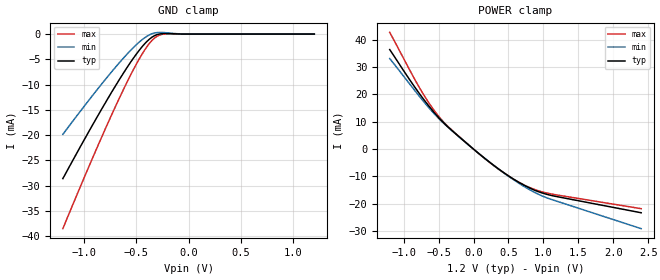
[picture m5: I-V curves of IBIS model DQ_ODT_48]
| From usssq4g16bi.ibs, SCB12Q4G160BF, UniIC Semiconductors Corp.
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|   Model DQ_ODT_48
[Model] DQ_ODT_48
Model_type Input
Polarity   Non-Inverting
Enable   Active-High
Vinl =  8.300E-01
Vinh =  9.700E-01
C_comp   7.893E-13   7.832E-13   8.052E-13
C_comp_power_clamp   2.190E-13   2.022E-13   2.435E-13
C_comp_gnd_clamp   5.703E-13   5.617E-13   5.809E-13
[Model Spec]
Vinh   9.700E-01   9.250E-01   1.015E+00
Vinl   8.300E-01   7.850E-01   8.750E-01
[Temperature Range]   45.000   95.000   -40.000
[Voltage Range]   1.200E+00   1.140E+00   1.260E+00
[C Comp Corner]
C_comp_power_clamp   2.190E-13   2.022E-13   2.435E-13
C_comp_gnd_clamp   5.703E-13   5.809E-13   5.617E-13
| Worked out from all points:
|   GND clamp passes 1 mA (typ) near -0.37 V on its own axis
|   POWER clamp passes 1 mA (typ) near -0.05 V on its own axis
[GND_clamp]
|Voltage   I(typ)   I(min)   I(max)
-1.2V     -28.63mA   -19.87mA   -38.54mA
-875mV    -16.5mA    -11.07mA   -22.57mA
-750mV    -12.06mA   -7.865mA   -16.71mA
-625mV    -7.836mA   -4.834mA   -11.13mA
-525mV    -4.725mA   -2.631mA   -6.977mA
-450mV    -2.664mA   -1.214mA   -4.181mA
-375mV    -1.027mA   -166uA     -1.874mA
-325mV    -315.4uA   217.4uA    -786.6uA
-275mV    28.27uA    334.2uA    -178.9uA
-200mV    103.9uA    241.9uA    49.02uA
-25mV     0A         0A         0A
1.2V      0A         0A         0A
[POWER_clamp]
|Voltage   I(typ)   I(min)   I(max)
-1.2V     36.4mA     33.1mA     42.68mA
-775mV    20.3mA     19.29mA    22.5mA
-625mV    15.29mA    14.69mA    16.38mA
-500mV    11.54mA    11.24mA    12.04mA
-375mV    8.324mA    8.207mA    8.507mA
-125mV    2.721mA    2.687mA    2.776mA
150mV     -3.161mA   -3.14mA    -3.216mA
400mV     -8.009mA   -8.069mA   -8.075mA
575mV     -11mA      -11.23mA   -11mA
725mV     -13.22mA   -13.68mA   -13.11mA
1V        -16.17mA   -17.31mA   -15.75mA
2.4V      -23.26mA   -29.08mA   -21.77mA
